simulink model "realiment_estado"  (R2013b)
settings: Solver=ode45  StartTime=0.0  StopTime=2  RelTol=1e-3
undefined symbols (not defined in the file): den_s, kp, kv, num_s, ts

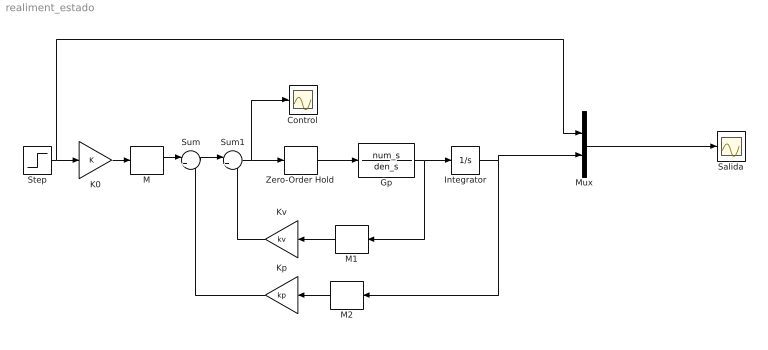
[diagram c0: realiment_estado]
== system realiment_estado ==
  Control : Scope
  Gp : TransferFcn  Numerator=num_s  Denominator=den_s
  Integrator : Integrator
  K0 : Gain  SampleTime=ts
  Kp : Gain  Gain=kp  SampleTime=ts
  Kv : Gain  Gain=kv  SampleTime=ts
  M : DiscreteTransferFcn  Numerator=1  Denominator=1  SampleTime=ts
  M1 : DiscreteTransferFcn  Numerator=1  Denominator=1  SampleTime=ts
  M2 : DiscreteTransferFcn  Numerator=1  Denominator=1  SampleTime=ts
  Mux : Mux  Inputs=2
  Salida : Scope
  Step : Step  Time=0  SampleTime=0
  Sum : Sum  Inputs=|+-
  Sum1 : Sum  Inputs=|+-
  Zero-Order Hold : ZeroOrderHold  SampleTime=ts
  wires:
  Step/1 -> Mux/1, K0/1
  M/1 -> Sum/1
  Mux/1 -> Salida/1
  Sum/1 -> Sum1/1
  Sum1/1 -> Zero-Order Hold/1, Control/1
  Zero-Order Hold/1 -> Gp/1
  Gp/1 -> Integrator/1, M1/1
  Integrator/1 -> Mux/2, M2/1
  M1/1 -> Kv/1
  M2/1 -> Kp/1
  Kv/1 -> Sum1/2
  Kp/1 -> Sum/2
  K0/1 -> M/1
